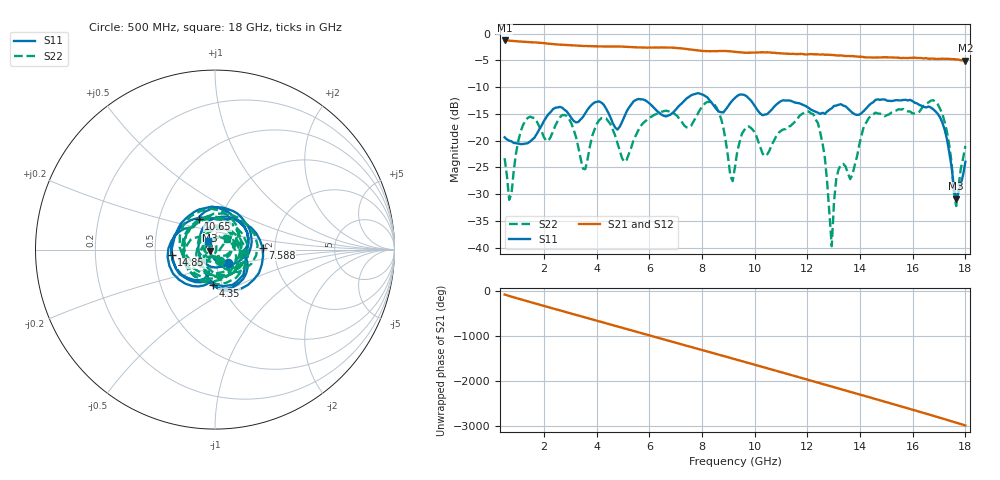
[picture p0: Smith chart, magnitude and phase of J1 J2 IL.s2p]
!Agilent Technologies,N5230A,MY45001360,A.07.50.67
!Agilent N5230A: A.07.50.67
!Date: Tuesday, April 16, 2024 17:32:22
!Correction: S11(Full 2 Port(1,2))
!S21(Full 2 Port(1,2))
!S12(Full 2 Port(1,2))
!S22(Full 2 Port(1,2))
!S2P File: Measurements: S11, S21, S12, S22:
# Hz S  dB  R 50
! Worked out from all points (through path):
!   201 points, 500 MHz to 18 GHz, reference 50 ohm
!   highest |S21| = -1.29 dB at 500 MHz (marker M1); lowest = -5.1 dB at 18 GHz (marker M2)
!   group delay of S21, straight-line fit = 458 ps
!   lowest |S11| = -30.8 dB at 17.65 GHz (marker M3), VSWR 1.06, Z = 47.3 - j0.639 ohm
!   |S11| at or under -10 dB: start of sweep to end of sweep
!   |S22| runs from -39.7 to -12.5 dB; largest |S21 - S12| = 0.0076
!   S11 on the Smith chart (normalised r, x): 500 MHz: 1.15, -0.18; 4.35 GHz: 0.90, -0.38; 7.588 GHz: 1.72, +0.04; 10.65 GHz: 0.79, +0.28; 14.85 GHz: 0.61, -0.04; 18 GHz: 0.92, +0.09
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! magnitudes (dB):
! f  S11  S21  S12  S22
! 500 MHz  -19.4  -1.3  -1.3  -23.3
! 675 MHz  -20.0  -1.3  -1.3  -31.1
! 1.288 GHz  -20.5  -1.5  -1.6  -16.3
! 2.775 GHz  -14.2  -2.1  -2.1  -15.2
! 3.475 GHz  -15.6  -2.3  -2.3  -25.2
! 4.35 GHz  -14.0  -2.4  -2.4  -15.8
! 5.05 GHz  -15.5  -2.5  -2.5  -24.0
! 6.362 GHz  -14.8  -2.6  -2.6  -14.8
! 7.588 GHz  -11.5  -3.0  -3.0  -17.2
! 8.375 GHz  -13.0  -3.3  -3.3  -12.8
! 9.25 GHz  -12.0  -3.4  -3.4  -24.9
! 9.688 GHz  -11.7  -3.6  -3.6  -17.5
! 10.65 GHz  -14.2  -3.6  -3.6  -20.7
! 12.22 GHz  -14.4  -3.9  -3.9  -15.1
! 12.66 GHz  -15.0  -4.0  -3.9  -23.2
! 12.93 GHz  -14.0  -4.0  -4.0  -39.7
! 13.19 GHz  -13.3  -4.1  -4.1  -25.3
! 14.85 GHz  -12.3  -4.4  -4.5  -15.1
! 15.11 GHz  -12.6  -4.5  -4.4  -15.1
! 16.95 GHz  -15.0  -4.7  -4.7  -13.2
! 17.65 GHz  -30.8  -4.8  -4.8  -32.2
! 18 GHz  -24.0  -5.1  -5.1  -21.0
